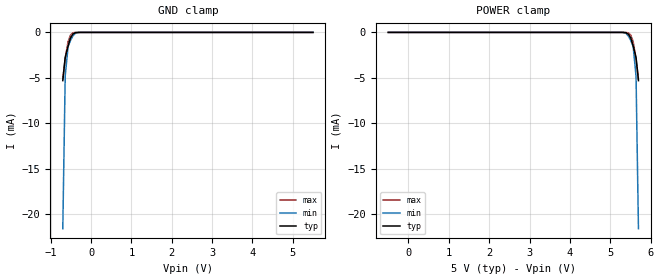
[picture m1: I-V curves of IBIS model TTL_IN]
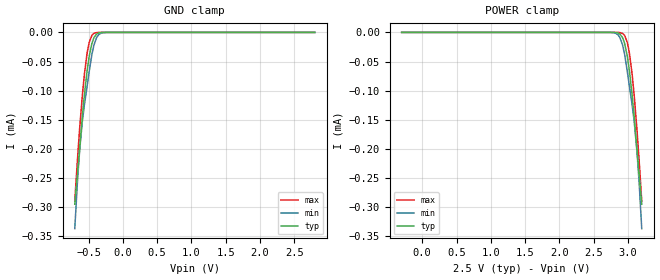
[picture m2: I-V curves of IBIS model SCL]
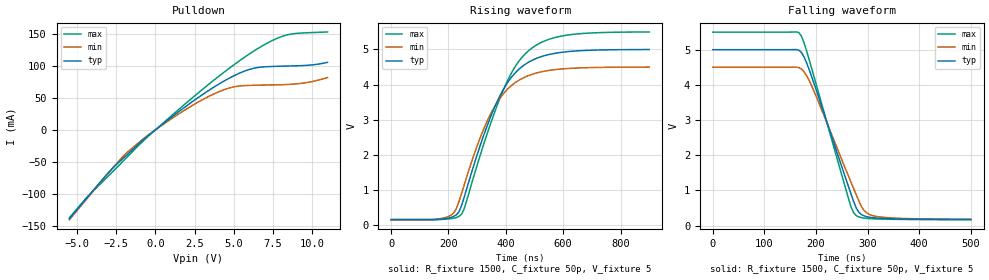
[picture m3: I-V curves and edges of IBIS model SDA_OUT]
[IBIS Ver]   3.2
[Comment Char]   |_char
[File name]   pca9530_5v.ibs
[File Rev]   1
[Date]   Nov 19, 2008 3:45:29 PM
[Source]
Generated by Seshadri Venkataramanan using IBIS Toolkit at NXP Tempe
[Notes]
[Disclaimer]
(C) Copyright 2007 NXP Semiconductors
All rights reserved
NXP Semiconductors (NXP) does not warrant that this model and any other
accompanying information (Model) accurately or fully represents the
operating characteristics and specifications of the semiconductor
products to which the Model relates.  Moreover, the Model is furnished
on an "as is" and with "all faults" basis, and without support or
warranty of any kind.  NXP disclaims all warranties, whether expressed
or implied or statutory, including without limitation all implied
warranties of non-infringement, merchantability and fitness for any
purpose, and those arising from a course of dealing or usage of trade.
NXP does not convey any license under its or any third party's patents,
copyrights or other intellectual property or proprietary rights.
You and your company assume any and all risks and liability arising out
of the application or use of the Model.
In no event shall NXP be liable for any direct, indirect, special,
consequential or incidental damages, however caused, whether in
warranty, contract or tort (including negligence), strict liability or
other legal theory, including, without limitation, for lost profits,
business interruption, or corruption or loss of data or information,
arising out of or in connection with the use of or the inability to use
the Model, even if NXP has been advised of the possibility of such
damages.
NXP provides the Model as a courtesy to our customers. You and your
company shall not distribute, convey, sell, or give the Model to anyone
else without receiving prior written permission from NXP.
NXP reserves the right to make changes without notice to the Model to
improve reliability, function, or design.
Please be aware that your receipt and subsequent use of the Model shall
serve as acceptance of these terms and conditions.  If you do not
accept these terms, return or destroy the Model immediately.
[Copyright]
2008
[Component]   PCA9530D
Si_location Pin
Timing_location Pin
[Manufacturer]   NXP Semiconductors
[Package]
R_pkg   4.81E-02   4.14E-02   5.47E-02
L_pkg   1.88E-09   1.54E-09   2.21E-09
C_pkg   4.49E-13   4.17E-13   4.81E-13
[Pin] signal_name   model_name   R_pin   L_pin   C_pin
1   A0   TTL_IN   5.47E-02  2.21E-09  4.81E-13
2   LED0   LED_OUT   4.14E-02  1.54E-09  4.20E-13
3   LED1   LED_OUT   4.14E-02  1.55E-09  4.20E-13
4   Vss   GND   5.47E-02  2.21E-09  4.80E-13
5   RESETb   TTL_IN   5.47E-02  2.21E-09  4.78E-13
6   SCL   SCL   4.14E-02  1.55E-09  4.17E-13
7   SDA   SDA   4.14E-02  1.54E-09  4.17E-13
8   VDD   POWER   5.47E-02  2.21E-09  4.79E-13
[Component]   PCA9530DP
Si_location Pin
Timing_location Pin
[Manufacturer]   NXP Semiconductors
[Package]
R_pkg   33.7m   30.1m   37.3m
L_pkg   1.74n   1.67n   1.81n
C_pkg   0.428p   0.422p   0.434p
[Pin] signal_name   model_name   R_pin   L_pin   C_pin
1   A0   TTL_IN   37.3m   1.81nH   0.428pF
2   LED0   LED_OUT   30.1m   1.67nH   0.422pF
3   LED1   LED_OUT   30.1m   1.67nH   0.428pF
4   Vss   GND   37.3m   1.81nH   0.434pF
5   RESETb   TTL_IN   37.3m   1.81nH   0.428pF
6   SCL   SCL   30.1m   1.67nH   0.422pF
7   SDA   SDA   30.1m   1.67nH   0.428pF
8   VDD   POWER   37.3m   1.81nH   0.434pF
[Model Selector]   SDA
SDA_IN   SDA Input
SDA_OUT   SDA output
| Models and submodels in the file (5): TTL_IN (Input), SCL (Input), SDA_OUT (Open_drain), LED_OUT (Open_drain), SDA_IN (Input)
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[Model]   TTL_IN
Model_type Input
Vinh=3.5
Vinl=1.5
C_comp   1.73p   1.7p   1.75p
[Temperature Range] 27   85   -40
[Voltage Range]   5   4.5   5.5
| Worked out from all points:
|   GND clamp passes 1 mA (typ) near -0.54 V on its own axis
[GND Clamp]
-700mV    -5.302mA   -21.58mA   -5.122mA
-640mV    -2.761mA   -4.801mA   -2.859mA
-570mV    -1.517mA   -1.6mA     -1.043mA
-510mV    -627uA     -899.4uA   -296.8uA
-450mV    -185.2uA   -388.2uA   -49.68uA
-390mV    -35.59uA   -105.7uA   -5.169uA
-200mV    -27.28nA   -200nA     -811.9pA
5.5V      106.9pA    399pA      72.28pA
[POWER Clamp]
-500mV    106.9pA    399pA      72.28pA
5.2V      -27.28nA   -200nA     -811.9pA
5.39V     -35.59uA   -105.7uA   -5.169uA
5.45V     -185.2uA   -388.2uA   -49.68uA
5.51V     -627uA     -899.4uA   -296.8uA
5.57V     -1.517mA   -1.6mA     -1.043mA
5.64V     -2.761mA   -4.801mA   -2.859mA
5.7V      -5.302mA   -21.58mA   -5.122mA
[Model]   SCL
Model_type Input
Vinh=1.75
Vinl=0.75
C_comp   3p   2.8p   3.2p
[Temperature Range] 27   85   -40
[Voltage Range]   2.5   2.2   2.8
[GND Clamp]
-700mV    -295uA     -337uA     -289.5uA
-660mV    -241.9uA   -254.1uA   -216.6uA
-630mV    -200.9uA   -204uA     -166.8uA
-590mV    -145.3uA   -153.2uA   -108.4uA
-560mV    -107.6uA   -124.5uA   -71.97uA
-520mV    -65.58uA   -92.63uA   -35.3uA
-490mV    -41.22uA   -67.38uA   -17.26uA
-450mV    -18.67uA   -37.44uA   -5.001uA
-420mV    -8.79uA    -21.47uA   -1.619uA
-350mV    -920.5nA   -3.647uA   -77.68nA
-210mV    -3.652nA   -27.14nA   -101.2pA
2.8V      6.71pA     20.63pA    5.609pA
[POWER Clamp]
-300mV    6.71pA     20.63pA    5.609pA
2.71V     -3.652nA   -27.14nA   -101.2pA
2.85V     -920.5nA   -3.647uA   -77.68nA
2.92V     -8.79uA    -21.47uA   -1.619uA
2.95V     -18.67uA   -37.44uA   -5.001uA
2.99V     -41.22uA   -67.38uA   -17.26uA
3.02V     -65.58uA   -92.63uA   -35.3uA
3.06V     -107.6uA   -124.5uA   -71.97uA
3.09V     -145.3uA   -153.2uA   -108.4uA
3.13V     -200.9uA   -204uA     -166.8uA
3.16V     -241.9uA   -254.1uA   -216.6uA
3.2V      -295uA     -337uA     -289.5uA
[Model]   SDA_OUT
Model_type Open_drain
Vref=3.5
Vmeas=1.5
Rref=1.5k
Cref=50p
C_comp   4p   3.8p   4.2p
[Temperature Range] 27   85   -40
[Voltage Range]   5   4.5   5.5
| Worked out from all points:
|   slope of the pulldown table from 0 to 0.75 V, typ, clamps not added: 51.6 ohm
|   falling waveform, R_fixture 1500, C_fixture 50p, V_fixture 5: 20-80 % time 66.1ns typ, 71.7ns min, 61.6ns max; typ from 5 V to 0.17 V
|   rising waveform, R_fixture 1500, C_fixture 50p, V_fixture 5: 20-80 % time 137ns typ, 131ns min, 144ns max; typ from 0.165 V to 5 V
[Pulldown]
-5.5V     -139.3mA   -140.7mA   -137.7mA
-4.33V    -105mA     -106.3mA   -104.4mA
-3V       -66.8mA    -67.57mA   -72.08mA
-1.83V    -39.36mA   -35.82mA   -43.15mA
170mV     3.328mA    2.952mA    3.702mA
2.83V     52.21mA    44.85mA    59.77mA
4.33V     75.65mA    62.32mA    89.18mA
5.5V      90.09mA    68.95mA    110.4mA
6.5V      97.46mA    69.88mA    126.6mA
7.5V      99.27mA    70.36mA    140.2mA
8.67V     100.1mA    71.35mA    149.9mA
11V       105.7mA    81.89mA    153.3mA
[Falling Waveform]
R_fixture=1500
C_fixture=50p
V_fixture=5
V_fixture_min=4.5
V_fixture_max=5.5
0s        5V         4.5V       5.5V
166.7ns   4.988V     4.491V     5.488V
176.8ns   4.796V     4.373V     5.199V
191.9ns   4.22V      3.962V     4.453V
267.7ns   905.4mV    1.236V     538.6mV
277.8ns   503.6mV    878.3mV    284.8mV
282.8ns   381.6mV    703.4mV    245.8mV
292.9ns   276mV      434.2mV    213.2mV
313.1ns   219.5mV    270.4mV    190.7mV
500ns     170.2mV    175.7mV    166.3mV
[Rising Waveform]
R_fixture=1500
C_fixture=50p
V_fixture=5
V_fixture_min=4.5
V_fixture_max=5.5
0s        164.7mV    166.4mV    163.4mV
200ns     209.1mV    253.6mV    184mV
227.3ns   299.7mV    470.8mV    224.1mV
245.5ns   557.6mV    900.9mV    314.7mV
309.1ns   2.233V     2.457V     1.951V
363.6ns   3.408V     3.415V     3.275V
427.3ns   4.285V     4.024V     4.441V
490.9ns   4.689V     4.293V     5.039V
618.2ns   4.941V     4.461V     5.413V
900ns     4.998V     4.499V     5.498V
[Ramp]
R_load=1500
dV/dt_r   2.901E+0/1.029E-7   2.889E+0/9.862E-8   2.910E+0/1.069E-7
dV/dt_f   2.898E+0/6.547E-8   2.883E+0/7.862E-8   2.909E+0/5.570E-8
|[End   SDA_OUT
